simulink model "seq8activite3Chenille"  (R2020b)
settings: Solver=VariableStepAuto  StartTime=0.0  StopTime=10.0  RelTol=1e-3  EnableMultiTasking=on
undefined symbols (not defined in the file): C, chenille_Defaut_sldprt, deg, Desktop, eg, kg, m, mm, N, rad, s, Seq8ExpGrapheEtats, table_Defaut_sldprt, Users, X, Y, Z
libraries: sm_lib x11, nesl_utility x4

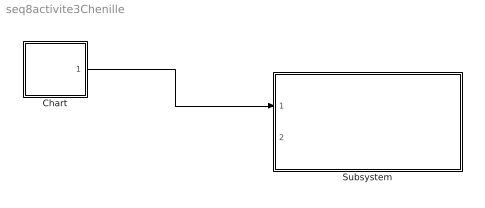
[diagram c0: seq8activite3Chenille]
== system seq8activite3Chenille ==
  Chart : Stateflow chart  TreatAsAtomicUnit=on
  Subsystem : Subsystem
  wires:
  Chart/1(AV) -> Subsystem/1(AV)

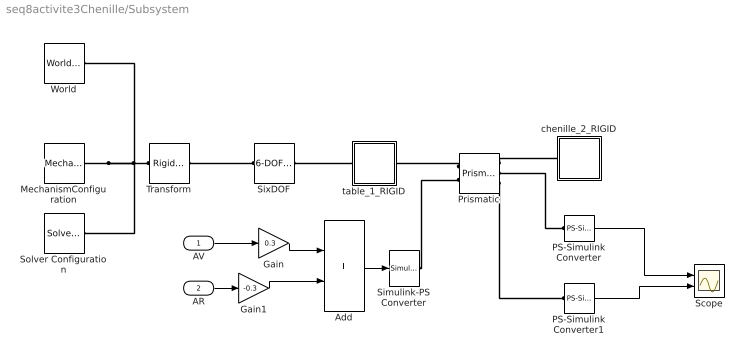
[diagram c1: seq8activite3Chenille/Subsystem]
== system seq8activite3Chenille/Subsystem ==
  AV : Inport
  AR : Inport  Port=2
  Add : Sum
  Gain : Gain  Gain=0.3
  Gain1 : Gain  Gain=-0.3
  MechanismConfiguration : sm_lib/Utilities/Mechanism Configuration  UniformGravity=Constant  GravityVector=[0 0 0]  GravityVectorUnits=m/s^2  GravityUnits=m/s^2  LinearizationDelta=0.001  JointModeTransitionNonlinearIterations=2
  PS-Simulink Converter : nesl_utility/PS-Simulink Converter  PhysicalDomain=network_engine_domain  SubClassName=ps_output  LeftPortType=input  RightPortType=output  PseudoPeriodic=off  Frequencies=[]  Unit=1  AffineConversion=off
  PS-Simulink Converter1 : nesl_utility/PS-Simulink Converter  PhysicalDomain=network_engine_domain  SubClassName=ps_output  LeftPortType=input  RightPortType=output  PseudoPeriodic=off  Frequencies=[]  Unit=1  AffineConversion=off
  Prismatic : sm_lib/Joints/Prismatic Joint  JointMode=Normal  SenseConstraintForce=off  SenseConstraintForceX=off  SenseConstraintForceY=off  SenseConstraintForceZ=off  SenseConstraintTorque=off  SenseConstraintTorqueX=off  SenseConstraintTorqueY=off  SenseConstraintTorqueZ=off  SenseTotalForce=off  SenseTotalForceX=off  SenseTotalForceY=off  SenseTotalForceZ=off  SenseTotalTorque=off  SenseTotalTorqueX=off  SenseTotalTorqueY=off  SenseTotalTorqueZ=off  CompositeWrenchDir=FollowerOnBase  CompositeWrenchFrame=BaseFrame  EquilibriumPosition=0  EquilibriumPositionUnits=m  SpringStiffness=0  SpringStiffnessUnits=N/m  DampingCoefficient=2  DampingCoefficientUnits=s*N/m  TorqueActuationMode=InputTorque  MotionActuationMode=ComputedMotion  SensePosition=on  SenseVelocity=on  SenseAcceleration=off  SenseTorqueForce=off  SenseLowerLimitTorqueForce=off  SenseUpperLimitTorqueForce=off  LowerLimitSpecify=off  LowerLimitBound=-1  LowerLimitBoundUnits=m  LowerLimitStiffness=1e6  LowerLimitStiffnessUnits=N/m  LowerLimitDamping=1e3  LowerLimitDampingUnits=N/(m/s)  LowerLimitTransitionRegionWidth=1e-4  LowerLimitTransitionRegionWidthUnits=m  UpperLimitSpecify=off  UpperLimitBound=1  UpperLimitBoundUnits=m  UpperLimitStiffness=1e6  UpperLimitStiffnessUnits=N/m  UpperLimitDamping=1e3  UpperLimitDampingUnits=N/(m/s)  UpperLimitTransitionRegionWidth=1e-4  UpperLimitTransitionRegionWidthUnits=m  PositionTargetSpecify=on  PositionTargetPriority=Low  PositionTargetValue=0  PositionTargetValueUnits=m  VelocityTargetSpecify=off  VelocityTargetPriority=High  VelocityTargetValue=0  VelocityTargetValueUnits=m/s
  Scope : Scope  NumInputPorts=2
  Simulink-PS Converter : nesl_utility/Simulink-PS Converter  PhysicalDomain=network_engine_domain  SubClassName=ps_input  LeftPortType=input  RightPortType=output  PseudoPeriodic=off  Frequencies=[]  NoiseDistribution=none  NoiseParameters=[]  Unit=1  AffineConversion=off  FilteringAndDerivatives=zero  SimscapeFilterOrder=1  InputFilterTimeConstant=0.001  UdotUserProvided=1
  SixDOF : sm_lib/Joints/6-DOF Joint  JointMode=Normal  SenseConstraintForce=off  SenseConstraintForceX=off  SenseConstraintForceY=off  SenseConstraintForceZ=off  SenseConstraintTorque=off  SenseConstraintTorqueX=off  SenseConstraintTorqueY=off  SenseConstraintTorqueZ=off  SenseTotalForce=off  SenseTotalForceX=off  SenseTotalForceY=off  SenseTotalForceZ=off  SenseTotalTorque=off  SenseTotalTorqueX=off  SenseTotalTorqueY=off  SenseTotalTorqueZ=off  CompositeWrenchDir=FollowerOnBase  CompositeWrenchFrame=BaseFrame  PxEquilibriumPosition=0  PxEquilibriumPositionUnits=m  PxSpringStiffness=0  PxSpringStiffnessUnits=N/m  PxDampingCoefficient=0  PxDampingCoefficientUnits=s*N/m  PxTorqueActuationMode=NoTorque  PxMotionActuationMode=ComputedMotion  PxSensePosition=off  PxSenseVelocity=off  PxSenseAcceleration=off  PxSenseTorqueForce=off  PxSenseLowerLimitTorqueForce=off  PxSenseUpperLimitTorqueForce=off  PxLowerLimitSpecify=off  PxLowerLimitBound=-1  PxLowerLimitBoundUnits=m  PxLowerLimitStiffness=1e6  PxLowerLimitStiffnessUnits=N/m  PxLowerLimitDamping=1e3  PxLowerLimitDampingUnits=N/(m/s)  PxLowerLimitTransitionRegionWidth=1e-4  PxLowerLimitTransitionRegionWidthUnits=m  PxUpperLimitSpecify=off  PxUpperLimitBound=1  PxUpperLimitBoundUnits=m  PxUpperLimitStiffness=1e6  PxUpperLimitStiffnessUnits=N/m  PxUpperLimitDamping=1e3  PxUpperLimitDampingUnits=N/(m/s)  PxUpperLimitTransitionRegionWidth=1e-4  PxUpperLimitTransitionRegionWidthUnits=m  PxPositionTargetSpecify=off  PxPositionTargetPriority=High  PxPositionTargetValue=0  PxPositionTargetValueUnits=m  PxVelocityTargetSpecify=off  PxVelocityTargetPriority=High  PxVelocityTargetValue=0  PxVelocityTargetValueUnits=m/s  PyEquilibriumPosition=0  PyEquilibriumPositionUnits=m  PySpringStiffness=0  PySpringStiffnessUnits=N/m  PyDampingCoefficient=0  PyDampingCoefficientUnits=s*N/m  PyTorqueActuationMode=NoTorque  PyMotionActuationMode=ComputedMotion  PySensePosition=off  PySenseVelocity=off  PySenseAcceleration=off  PySenseTorqueForce=off  PySenseLowerLimitTorqueForce=off  PySenseUpperLimitTorqueForce=off  PyLowerLimitSpecify=off  PyLowerLimitBound=-1  PyLowerLimitBoundUnits=m  PyLowerLimitStiffness=1e6  PyLowerLimitStiffnessUnits=N/m  PyLowerLimitDamping=1e3  PyLowerLimitDampingUnits=N/(m/s)  PyLowerLimitTransitionRegionWidth=1e-4  PyLowerLimitTransitionRegionWidthUnits=m  PyUpperLimitSpecify=off  PyUpperLimitBound=1  PyUpperLimitBoundUnits=m  PyUpperLimitStiffness=1e6  PyUpperLimitStiffnessUnits=N/m  PyUpperLimitDamping=1e3  PyUpperLimitDampingUnits=N/(m/s)  PyUpperLimitTransitionRegionWidth=1e-4  PyUpperLimitTransitionRegionWidthUnits=m  PyPositionTargetSpecify=off  PyPositionTargetPriority=High  PyPositionTargetValue=0  PyPositionTargetValueUnits=m  PyVelocityTargetSpecify=off  PyVelocityTargetPriority=High  PyVelocityTargetValue=0  PyVelocityTargetValueUnits=m/s  PzEquilibriumPosition=0  PzEquilibriumPositionUnits=m  PzSpringStiffness=0  PzSpringStiffnessUnits=N/m  PzDampingCoefficient=0  PzDampingCoefficientUnits=s*N/m  PzTorqueActuationMode=NoTorque  PzMotionActuationMode=ComputedMotion  PzSensePosition=off  PzSenseVelocity=off  PzSenseAcceleration=off  PzSenseTorqueForce=off  PzSenseLowerLimitTorqueForce=off  PzSenseUpperLimitTorqueForce=off  PzLowerLimitSpecify=off  PzLowerLimitBound=-1  PzLowerLimitBoundUnits=m  PzLowerLimitStiffness=1e6  PzLowerLimitStiffnessUnits=N/m  PzLowerLimitDamping=1e3  PzLowerLimitDampingUnits=N/(m/s)  PzLowerLimitTransitionRegionWidth=1e-4  PzLowerLimitTransitionRegionWidthUnits=m  PzUpperLimitSpecify=off  PzUpperLimitBound=1  PzUpperLimitBoundUnits=m  PzUpperLimitStiffness=1e6  PzUpperLimitStiffnessUnits=N/m  PzUpperLimitDamping=1e3  PzUpperLimitDampingUnits=N/(m/s)  PzUpperLimitTransitionRegionWidth=1e-4  PzUpperLimitTransitionRegionWidthUnits=m  PzPositionTargetSpecify=off  PzPositionTargetPriority=High  PzPositionTargetValue=0  PzPositionTargetValueUnits=m  PzVelocityTargetSpecify=off  PzVelocityTargetPriority=High  PzVelocityTargetValue=0  PzVelocityTargetValueUnits=m/s  SphDefPosRotationMethod=None  SphDefPosRotationAngleUnits=deg  SphDefPosRotationStandardAxis=+Z  SphDefPosRotationAngle=0.0  SphDefPosRotationArbitraryAxis=[0 0 1]  SphDefPosFollAlignAxisA=+X  SphDefPosBaseAlignAxisA=+Y  SphDefPosFollAlignAxisB=+Y  SphDefPosBaseAlignAxisB=+Z  SphDefPosRotationSequenceAxes=FollowerAxes  SphDefPosRotationSequence=XYX  SphDefPosRotationSequenceAngles=[0 0 0]  SphDefPosRotationSequenceAnglesUnits=deg  SphDefPosRotationMatrix=[1 0 0; 0 1 0; 0 0 1]  SphEqPosRotationMethod=None  SphEqPosRotationAngleUnits=deg  SphEqPosRotationStandardAxis=+Z  SphEqPosRotationAngle=0.0  SphEqPosRotationArbitraryAxis=[0 0 1]  SphEqPosFollAlignAxisA=+X  SphEqPosBaseAlignAxisA=+Y  SphEqPosFollAlignAxisB=+Y  SphEqPosBaseAlignAxisB=+Z  SphEqPosRotationSequenceAxes=FollowerAxes  SphEqPosRotationSequence=XYX  SphEqPosRotationSequenceAngles=[0 0 0]  SphEqPosRotationSequenceAnglesUnits=deg  SphEqPosRotationMatrix=[1 0 0; 0 1 0; 0 0 1]  SphSpringStiffness=0  SphSpringStiffnessUnits=m*N/rad  SphDampingCoefficient=0  SphDampingCoefficientUnits=m*s*N/rad  SphActuateTorqueX=off  SphActuateTorqueY=off  SphActuateTorqueZ=off  SphActuateTorque=off  SphTorqueActuationMode=NoTorque  SphMotionActuationMode=ComputedMotion  SphActuationFrame=BaseFrame  SphSensePosition=off  SphSenseVelocityX=off  SphSenseVelocityY=off  SphSenseVelocityZ=off  SphSenseVelocity=off  SphSenseAccelerationX=off  SphSenseAccelerationY=off  SphSenseAccelerationZ=off  SphSenseAcceleration=off  SphSenseTorqueX=off  SphSenseTorqueY=off  SphSenseTorqueZ=off  SphSenseTorqueForce=off  SphSenseLowerLimitTorqueMag=off  SphSenseUpperLimitTorqueMag=off  SphSensingFrame=FollowerFrame  SphLowerLimitSpecify=off  SphLowerLimitBound=15  SphLowerLimitBoundUnits=deg  SphLowerLimitStiffness=1e4  SphLowerLimitStiffnessUnits=N*m/deg  SphLowerLimitDamping=10  SphLowerLimitDampingUnits=N*m/(deg/s)  SphLowerLimitTransitionRegionWidth=0.1  SphLowerLimitTransitionRegionWidthUnits=deg  SphUpperLimitSpecify=off  SphUpperLimitBound=45  SphUpperLimitBoundUnits=deg  SphUpperLimitStiffness=1e4  SphUpperLimitStiffnessUnits=N*m/deg  SphUpperLimitDamping=10  SphUpperLimitDampingUnits=N*m/(deg/s)  SphUpperLimitTransitionRegionWidth=0.1  SphUpperLimitTransitionRegionWidthUnits=deg  SphPositionTargetRotationMethod=None  SphPositionTargetRotationAngleUnits=deg  SphPositionTargetRotationStandardAxis=+Z  SphPositionTargetRotationAngle=0.0  SphPositionTargetRotationArbitraryAxis=[0 0 1]  SphPositionTargetFollAlignAxisA=+X  SphPositionTargetBaseAlignAxisA=+Y  SphPositionTargetFollAlignAxisB=+Y  SphPositionTargetBaseAlignAxisB=+Z  SphPositionTargetRotationSequenceAxes=FollowerAxes  SphPositionTargetRotationSequence=XYX  SphPositionTargetRotationSequenceAngles=[0 0 0]  SphPositionTargetRotationSequenceAnglesUnits=deg  SphPositionTargetRotationMatrix=[1 0 0; 0 1 0; 0 0 1]  SphPositionTargetSpecify=off  SphPositionTargetPriority=High  SphVelocityTargetValue=[0 0 0]  SphVelocityTargetValueUnits=deg/s  SphVelocityTargetSpecify=off  SphVelocityTargetPriority=High  SphVelocityTargetInFollowerFrame=on
  Solver Configuration : nesl_utility/Solver Configuration  PhysicalDomain=network_engine_domain  SubClassName=solver  LeftPortType=input  RightPortType=generic  Tones=[]  Harmonics=[]  SimulateNoise=off  Profile=off  UseLocalSampling=off  EnableSwitchedLinearOptims=on  FrequencyDomain=off  UseCCode=off  RelTol=0.001  AbsTol=1e-06  MinStep=1e-09  ToWorkspace=off  RevertToSquareIcSolve=off  NumHomotopyIterations=100  PhasorMode=off  PhasorModeNumHarmonics=1  DoDC=off  ResidualTolerance=1e-09  UseLocalSolver=off  LocalSolverChoice=NE_BACKWARD_EULER_ADVANCER  LocalSolverSampleTime=0.001  DoFixedCost=off  MaxNonlinIter=3  MaxModeIter=2  ComputeImpulses=off  ImpulseIterations=2  LinearAlgebra=Sparse  EquationFormulation=NE_TIME_EF  DelaysMemoryBudget=1024  AutomaticFiltering=on  FilteringTimeConstant=0.001  PartitionStorageMethod=AS_NEEDED  PartitionMemoryBudget=1024  PartitionMethod=FAST
  Transform : sm_lib/Frames and Transforms/Rigid Transform  TranslationMethod=Cartesian  TranslationStandardOffset=0  TranslationLengthUnit=mm  TranslationStandardAxis=+Z  TranslationCartesianOffset=[-1347.9501879485856 -195.69217875039209 195.88319786837215]  TranslationROffset=0  TranslationROffsetUnits=m  TranslationZOffset=0  TranslationZOffsetUnits=m  TranslationThetaOffset=0  TranslationThetaOffsetUnits=deg  RotationMethod=None  RotationAngleUnits=deg  RotationStandardAxis=+Z  RotationAngle=0.0  RotationArbitraryAxis=[0 0 1]  FollAlignAxisA=+X  BaseAlignAxisA=+Y  FollAlignAxisB=+Y  BaseAlignAxisB=+Z  RotationSequenceAxes=FollowerAxes  RotationSequence=XYX  RotationSequenceAngles=[0 0 0]  RotationSequenceAnglesUnits=deg  RotationMatrix=[1 0 0; 0 1 0; 0 0 1]
  World : sm_lib/Frames and Transforms/World Frame
  chenille_2_RIGID : Subsystem
  table_1_RIGID : Subsystem
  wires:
  AV/1 -> Gain/1
  PS-Simulink Converter/1 -> Scope/1
  PS-Simulink Converter1/1 -> Scope/2
  Gain/1 -> Add/1
  Add/1 -> Simulink-PS Converter/1
  AR/1 -> Gain1/1
  Gain1/1 -> Add/2
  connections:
  Transform/LConn1 -- MechanismConfiguration/RConn1 -- Solver Configuration/RConn1 -- World/RConn1
  Prismatic/LConn1 -- table_1_RIGID/RConn1
  SixDOF/LConn1 -- Transform/RConn1
  Prismatic/RConn1 -- chenille_2_RIGID/LConn1
  SixDOF/RConn1 -- table_1_RIGID/LConn1
  Prismatic/RConn3 -- PS-Simulink Converter1/LConn1
  Simulink-PS Converter/RConn1 -- Prismatic/LConn2
  PS-Simulink Converter/LConn1 -- Prismatic/RConn2

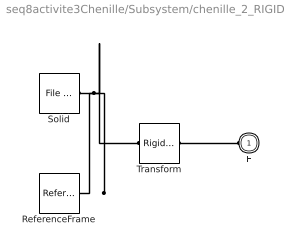
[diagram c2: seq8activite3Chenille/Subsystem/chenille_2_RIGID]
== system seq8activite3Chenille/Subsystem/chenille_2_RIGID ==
  ReferenceFrame : sm_lib/Frames and Transforms/Reference Frame
  Solid : sm_lib/Body Elements/File Solid  ExtGeomFileName=C:\Users\eg\Desktop\Seq8ExpGrapheEtats\chenille_Defaut_sldprt.STEP  UnitType=FromFile  ExtGeomFileUnits=m  StepReaderType=HEX  ExportConvexHullGeometry=off  InertiaType=Custom  Mass=0.97053981633974484  MassUnits=kg  CenterOfMass=[84.999999999999972 22.10257654274357 -39.999999999999993]  CenterOfMassUnits=mm  MomentsOfInertia=[1332.3789533957931 3262.3223254581671 2365.2995427325859]  MomentsOfInertiaUnits=kg*mm^2  ProductsOfInertia=[0 0 0]  ProductsOfInertiaUnits=kg*mm^2  BasedOnType=Density  Density=1000  DensityUnits=kg/(m^3)  DoExposeReferenceFrame=on  SerializedFrames=<Frames/>  GraphicType=FromGeometry  MarkerShape=Sphere  MarkerSize=10  GraphicVisPropType=SimpleVisualProperties  GraphicDiffuseColor=[0.792156862745098 0.81960784313725488 0.93333333333333335]  GraphicSpecularColor=[0.5 0.5 0.5 1.0]  GraphicAmbientColor=[0.15 0.15 0.15 1.0]  GraphicEmissiveColor=[0.0 0.0 0.0 1.0]  GraphicShininess=75  GraphicOpacity=1
  Transform : sm_lib/Frames and Transforms/Rigid Transform  TranslationMethod=Cartesian  TranslationStandardOffset=0  TranslationLengthUnit=mm  TranslationStandardAxis=+Z  TranslationCartesianOffset=[-1641.5934773244367 -10.000000000000085 50]  TranslationROffset=0  TranslationROffsetUnits=m  TranslationZOffset=0  TranslationZOffsetUnits=m  TranslationThetaOffset=0  TranslationThetaOffsetUnits=deg  RotationMethod=ArbitraryAxis  RotationAngleUnits=rad  RotationStandardAxis=+Z  RotationAngle=2.0943951023931953  RotationArbitraryAxis=[-0.57735026918962584 -0.57735026918962584 0.57735026918962584]  FollAlignAxisA=+X  BaseAlignAxisA=+Y  FollAlignAxisB=+Y  BaseAlignAxisB=+Z  RotationSequenceAxes=FollowerAxes  RotationSequence=XYX  RotationSequenceAngles=[0 0 0]  RotationSequenceAnglesUnits=deg  RotationMatrix=[1 0 0; 0 1 0; 0 0 1]
  F : PMIOPort  Side=Left
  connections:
  Solid/RConn1 -- ReferenceFrame/RConn1 -- Transform/LConn1
  Transform/RConn1 -- F/RConn1

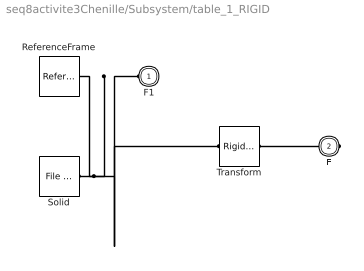
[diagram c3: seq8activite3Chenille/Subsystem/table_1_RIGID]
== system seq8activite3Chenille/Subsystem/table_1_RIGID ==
  ReferenceFrame : sm_lib/Frames and Transforms/Reference Frame
  Solid : sm_lib/Body Elements/File Solid  ExtGeomFileName=C:\Users\eg\Desktop\Seq8ExpGrapheEtats\table_Defaut_sldprt.STEP  UnitType=FromFile  ExtGeomFileUnits=m  StepReaderType=HEX  ExportConvexHullGeometry=off  InertiaType=Custom  Mass=8.9999999999999982  MassUnits=kg  CenterOfMass=[2999.9999999999995 5 -75]  CenterOfMassUnits=mm  MomentsOfInertia=[16949.999999999993 27016874.999999989 27000074.999999989]  MomentsOfInertiaUnits=kg*mm^2  ProductsOfInertia=[0 0 0]  ProductsOfInertiaUnits=kg*mm^2  BasedOnType=Density  Density=1000  DensityUnits=kg/(m^3)  DoExposeReferenceFrame=on  SerializedFrames=<Frames/>  GraphicType=FromGeometry  MarkerShape=Sphere  MarkerSize=10  GraphicVisPropType=SimpleVisualProperties  GraphicDiffuseColor=[0.792156862745098 0.81960784313725488 0.93333333333333335]  GraphicSpecularColor=[0.5 0.5 0.5 1.0]  GraphicAmbientColor=[0.15 0.15 0.15 1.0]  GraphicEmissiveColor=[0.0 0.0 0.0 1.0]  GraphicShininess=75  GraphicOpacity=1
  Transform : sm_lib/Frames and Transforms/Rigid Transform  TranslationMethod=Cartesian  TranslationStandardOffset=0  TranslationLengthUnit=mm  TranslationStandardAxis=+Z  TranslationCartesianOffset=[0 10.000000000000009 0]  TranslationROffset=0  TranslationROffsetUnits=m  TranslationZOffset=0  TranslationZOffsetUnits=m  TranslationThetaOffset=0  TranslationThetaOffsetUnits=deg  RotationMethod=ArbitraryAxis  RotationAngleUnits=rad  RotationStandardAxis=+Z  RotationAngle=2.0943951023931953  RotationArbitraryAxis=[-0.57735026918962584 -0.57735026918962584 0.57735026918962584]  FollAlignAxisA=+X  BaseAlignAxisA=+Y  FollAlignAxisB=+Y  BaseAlignAxisB=+Z  RotationSequenceAxes=FollowerAxes  RotationSequence=XYX  RotationSequenceAngles=[0 0 0]  RotationSequenceAnglesUnits=deg  RotationMatrix=[1 0 0; 0 1 0; 0 0 1]
  F1 : PMIOPort  Side=Left
  F : PMIOPort  Port=2  Side=Right
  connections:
  Solid/RConn1 -- ReferenceFrame/RConn1 -- Transform/LConn1 -- F1/RConn1
  Transform/RConn1 -- F/RConn1

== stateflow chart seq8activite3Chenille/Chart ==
  data: AV output
